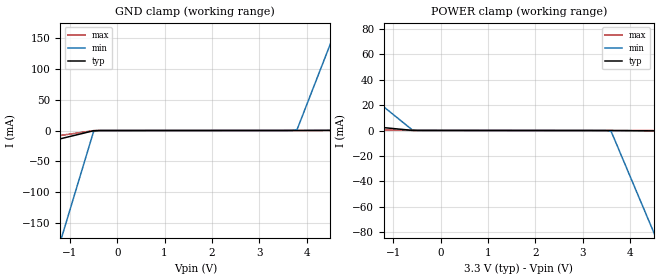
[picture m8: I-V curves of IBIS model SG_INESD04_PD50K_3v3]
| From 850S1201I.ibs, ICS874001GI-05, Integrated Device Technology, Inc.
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[Model] SG_INESD04_PD50K_3v3
Model_type   Input
Polarity   Non-Inverting
Vinl = 0.80V
Vinh = 2.2V
|   typ   min   max
C_comp   2pF   1.5pF   2.5pF
|   typ   min   max
[Voltage range]  3.3V   3.135V   3.456V
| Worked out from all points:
|   GND clamp passes 1 mA (typ) near -0.53 V on its own axis
|   POWER clamp passes 1 mA (typ) near -0.85 V on its own axis
[GND_clamp]
|Voltage   I(typ)   I(min)   I(max)
-3.3V     -52.25mA   -711.5mA   -31.55mA
-1.2V     -13.34mA   -179.1mA   -8.006mA
-1.1V     -11.49mA   -153.7mA   -6.884mA
-500mV    -368.1uA   -1.645mA   -156.4uA
-300mV    -6.904uA   -14.83uA   -5.752uA
3.6V      71.67uA    90.6uA     68.21uA
3.8V      78.53uA    1.463mA    72.01uA
4.6V      403.2uA    158.9mA    87.29uA
4.7V      443.8uA    178.6mA    89.2uA
6.6V      1.215mA    552.6mA    125.5uA
[POWER_clamp]
|Voltage   I(typ)   I(min)   I(max)
-3.3V     9.738mA    81.75mA    2.011mA
-600mV    119.1uA    404uA      81.23uA
3.4V      -1.989uA   -8.579uA   1.23uA
3.6V      -6.904uA   -691.8uA   -2.555uA
4.5V      -247.9uA   -80.18mA   -19.62uA
4.6V      -274.7uA   -89.02mA   -21.52uA
6.6V      -810.3uA   -265.7mA   -59.45uA
